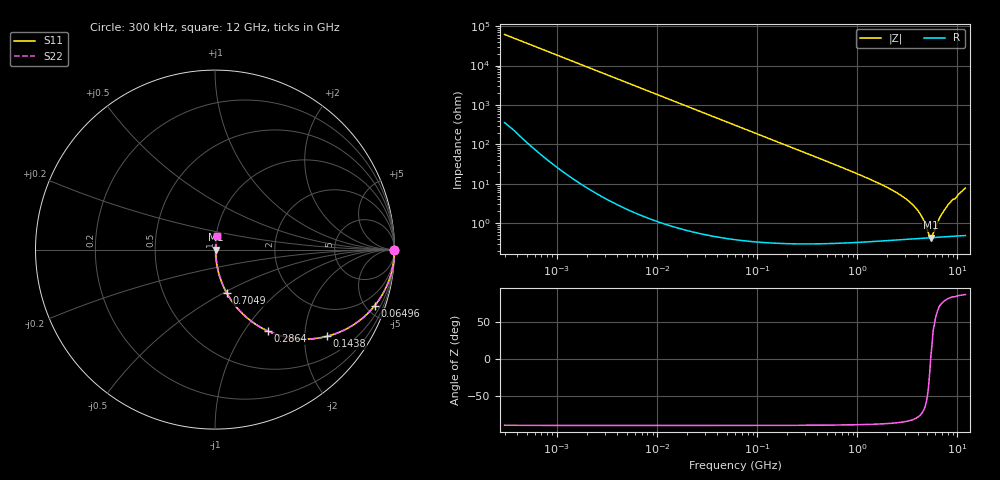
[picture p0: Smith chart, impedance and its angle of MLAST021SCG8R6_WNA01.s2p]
! MLAST021SCG8R6_WNA01  S-PARAMETER MODEL  ( General Type )
! Model Generated by TAIYO YUDEN Corporation (http://www.ty-top.com)
! Version 1.0
! TAIYO YUDEN Control No. 220901
! Copyright(c) 2022 TAIYO YUDEN CO.,LTD. All Rights Reserved.
! Product Description (link to TY-COMPAS)
! https://ds.yuden.co.jp/TYCOMPAS/or/detail?pn=MLAST021SCG8R6CWNA01&u=M
! Products Name : Multilayer Ceramic Capacitors
! Characteristics :
!  Capacitance : 8.6 pF , Rated Voltage : 25V , TCC : CG / C0G
!  Case Size : 0.25 x 0.125 / 0.0098 x 0.0049 [mm/inch] , Thickness : 0.125 / 0.0049 [mm/inch]
!  (Conditions: Temperature = 25 degC , DC Bias Current/Voltage = 0A / 0V)
! External Node Assignments :
!  1  o---| |---o  2
! GND o---------o GND
! Frequency Range : 0.3MHz  -  12000MHz  [ 401 STEP ]
# MHz S RI R 50
! Freq[MHz].  S11 Real  S11 Imag  S21 Real  S21 Imag  S12 Real  S12 Imag  S22 Real  S22 Imag
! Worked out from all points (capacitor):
!   401 points, 300 kHz to 12 GHz, reference 50 ohm
!   read as one part in series: C = 8.6 pF near 316.3 kHz
!   lowest |Z| = 428 mohm at 5.42 GHz (marker M1)
!   series resonance near 5.403 GHz, so ESL is about 100 pH
!   S11 on the Smith chart (normalised r, x): 300 kHz: open; 64.96 MHz: 1.01, -5.70; 143.8 MHz: 1.01, -2.57; 286.4 MHz: 1.01, -1.29; 704.9 MHz: 1.01, -0.52; 12 GHz: 1.01, +0.15
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0.3  1 -0.00162  1.2e-05 0.00162  1.2e-05 0.00162  1 -0.00162
1.769972  0.9999 -0.00956  0.0001 0.00956  0.0001 0.00956  0.9999 -0.00956
10.44266  0.9968 -0.0562  0.00321 0.0562  0.00321 0.0562  0.9968 -0.0562
26.39317  0.98 -0.1397  0.02 0.1397  0.02 0.1397  0.98 -0.1397
60  0.9046 -0.2932  0.0954 0.2932  0.0954 0.2932  0.9046 -0.2932
64.96309  0.89 -0.3123  0.11 0.3123  0.11 0.3123  0.89 -0.3123
96.65937  0.7852 -0.4098  0.2148 0.4098  0.2148 0.4098  0.7852 -0.4098
143.8206  0.6228 -0.4835  0.3772 0.4835  0.3772 0.4835  0.6228 -0.4835
202.9496  0.4535 -0.4962  0.5465 0.4962  0.5465 0.4962  0.4535 -0.4962
286.3882  0.2943 -0.4534  0.7057 0.4534  0.7057 0.4534  0.2943 -0.4534
353.9943  0.2145 -0.4077  0.7855 0.4077  0.7855 0.4077  0.2145 -0.4077
704.9044  0.065 -0.2405  0.935 0.2405  0.935 0.2405  0.065 -0.2405
2088.533  0.00919 -0.0744  0.9908 0.0744  0.9908 0.0744  0.00919 -0.0744
2947.191  0.00575 -0.0436  0.9943 0.0436  0.9943 0.0436  0.00575 -0.0436
3740.715  0.00465 -0.0255  0.9954 0.0255  0.9954 0.0255  0.00465 -0.0255
4385.161  0.00431 -0.0142  0.9957 0.0142  0.9957 0.0142  0.00431 -0.0142
5140.631  0.00423 -0.0033  0.9958 0.0033  0.9958 0.0033  0.00423 -0.0033
5420.343  0.00426 0.000212  0.9957 -0.000212  0.9957 -0.000212  0.00426 0.000212
5715.274  0.00431 0.00333  0.9957 -0.00333  0.9957 -0.00333  0.00431 0.00333
6699.894  0.00459 0.0135  0.9954 -0.0135  0.9954 -0.0135  0.00459 0.0135
7854.144  0.0052 0.0258  0.9948 -0.0258  0.9948 -0.0258  0.0052 0.0258
12000  0.0106 0.076  0.9894 -0.076  0.9894 -0.076  0.0106 0.076
